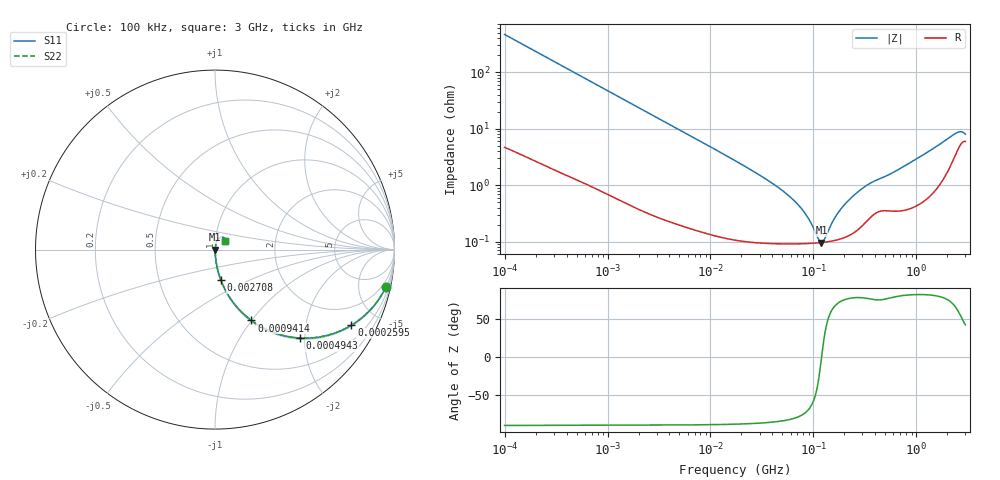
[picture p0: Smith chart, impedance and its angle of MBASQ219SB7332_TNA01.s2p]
! MBASQ219SB7332_TNA01  S-PARAMETER MODEL  ( Standard Model )
! Model Generated by TAIYO YUDEN Corporation (http://www.ty-top.com)
! Version 1.0
! TAIYO YUDEN Control No. 220601
! Copyright(c) 2013 TAIYO YUDEN CO.,LTD. All Rights Reserved.
! Product Description (link to TY-COMPAS)
! https://ds.yuden.co.jp/TYCOMPAS/or/detail?pn=MBASQ219SB7332KTNA01&u=M
! Products Name : Multilayer Ceramic Capacitors
! Characteristics :
!  Capacitance : 3300 [pF] , Rated Voltage : 250 [V] , TCC : X7R
!  Case Size : 2.0 x 1.25 / 0.079 x 0.049 [mm/inch] , Thickness : 0.85 / 0.033 [mm/inch]
!  (Conditions: Temperature = 25 [degC] , DC Bias Voltage = 0 [V])
! External Node Assignments :
!  1  o---| |---o  2
! GND o---------o GND
! Frequency Range : 100kHz  -  3GHz  [ 401 STEP ]
# MHZ S RI R 50
! Freq[MHz].  S11 Real  S11 Imag  S21 Real  S21 Imag  S12 Real  S12 Imag  S22 Real  S22 Imag
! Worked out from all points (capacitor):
!   401 points, 100 kHz to 3 GHz, reference 50 ohm
!   read as one part in series: C = 3.44 nF near 105.3 kHz
!   lowest |Z| = 96.9 mohm at 119.7 MHz (marker M1)
!   series resonance near 120.2 MHz, so ESL is about 510 pH
!   S11 on the Smith chart (normalised r, x): 100 kHz: 1.09, -9.23; 259.5 kHz: 1.04, -3.58; 494.3 kHz: 1.03, -1.89; 941.4 kHz: 1.01, -1.00; 2.708 MHz: 1.01, -0.35; 3 GHz: 1.12, +0.11
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0.1  0.9533 -0.2061  0.0467 0.2061  0.0467 0.2061  0.9533 -0.2061
0.167439  0.8818 -0.3173  0.1182 0.3173  0.1182 0.3173  0.8818 -0.3173
0.259498  0.7598 -0.4213  0.2402 0.4213  0.2402 0.4213  0.7598 -0.4213
0.494258  0.4722 -0.4926  0.5278 0.4926  0.5278 0.4926  0.4722 -0.4926
0.562235  0.4102 -0.4851  0.5898 0.4851  0.5898 0.4851  0.4102 -0.4851
0.941399  0.2029 -0.395  0.7971 0.395  0.7971 0.395  0.2029 -0.395
1.497078  0.0939 -0.2842  0.9061 0.2842  0.9061 0.2842  0.0939 -0.2842
2.708188  0.0324 -0.1688  0.9676 0.1688  0.9676 0.1688  0.0324 -0.1688
3.161081  0.0245 -0.146  0.9755 0.146  0.9755 0.146  0.0245 -0.146
17.7727  0.00175 -0.0264  0.9982 0.0264  0.9982 0.0264  0.00175 -0.0264
56.67997  0.000958 -0.00661  0.999 0.00661  0.999 0.00661  0.000958 -0.00661
77.22239  0.000934 -0.00367  0.9991 0.00367  0.9991 0.00367  0.000934 -0.00367
97.38194  0.000941 -0.00171  0.9991 0.00171  0.9991 0.00171  0.000941 -0.00171
110.7752  0.000955 -0.00066  0.999 0.00066  0.999 0.00066  0.000955 -0.00066
119.6798  0.000967 -3.75e-05  0.999 3.75e-05  0.999 3.75e-05  0.000967 -3.75e-05
129.3002  0.000983 0.000586  0.999 -0.000586  0.999 -0.000586  0.000983 0.000586
171.6802  0.00109 0.00295  0.9989 -0.00295  0.9989 -0.00295  0.00109 0.00295
222.1509  0.00131 0.00533  0.9987 -0.00533  0.9987 -0.00533  0.00131 0.00533
335.5313  0.00246 0.00979  0.9975 -0.00979  0.9975 -0.00979  0.00246 0.00979
547.5153  0.00372 0.015  0.9963 -0.015  0.9963 -0.015  0.00372 0.015
2378.954  0.0368 0.0692  0.9632 -0.0692  0.9632 -0.0692  0.0368 0.0692
3000  0.0583 0.0475  0.9417 -0.0475  0.9417 -0.0475  0.0583 0.0475
